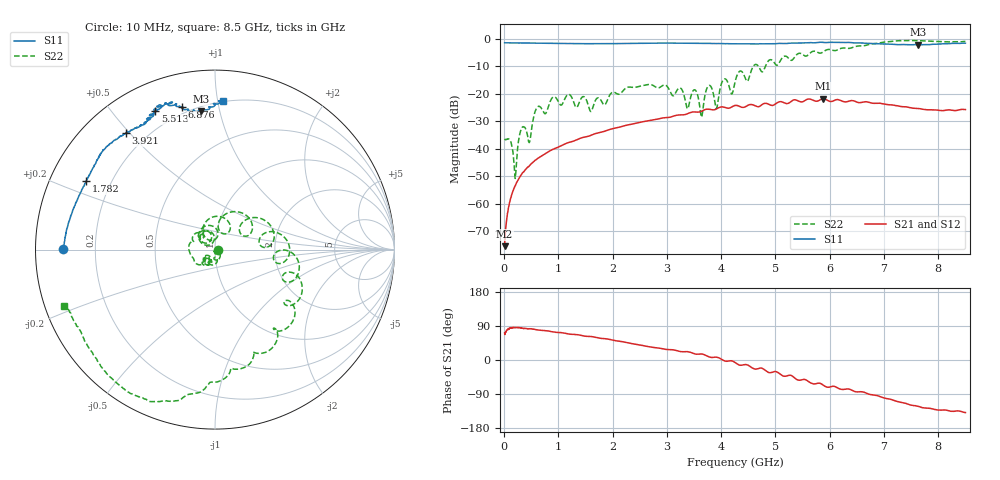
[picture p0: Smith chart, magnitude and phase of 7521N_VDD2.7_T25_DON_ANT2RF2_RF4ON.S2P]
!Agilent Technologies,E5071C,MY46417908,A.11.23
!Date: Thu Jul 30 15:13:54 2020
!Data & Calibration Information:
!Freq	S11:SOLT2(ON)	S21:SOLT2(ON)	S12:SOLT2(ON)	S22:SOLT2(ON)
!PortZ  Port1:50+j0  Port2:50+j0
!Above PortZ is port z conversion or system Z0 setting when saving the data.
!When reading, reference impedance value at option line is always used.
# Hz S dB R 50
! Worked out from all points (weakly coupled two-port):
!   1601 points, 10 MHz to 8.5 GHz, reference 50 ohm
!   highest |S21| = -21.85 dB at 5.879 GHz (marker M1); lowest = -75.5 dB at 10 MHz (marker M2)
!   lowest |S11| = -2.2 dB at 7.624 GHz (marker M3), VSWR 7.90, Z = 11.3 + j43.8 ohm
!   |S11| at or under -10 dB: nowhere
!   |S22| runs from -50.9 to -0.6 dB; largest |S21 - S12| = 0.00077
!   S11 on the Smith chart (normalised r, x): 10 MHz: 0.08, +0.00; 1.782 GHz: 0.11, +0.25; 3.921 GHz: 0.13, +0.49; 5.513 GHz: 0.12, +0.65; 6.876 GHz: 0.17, +0.78; 8.5 GHz: 0.20, +1.04
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1e7  -1.45 179.9  -75.50 71.1  -75.74 70.6  -36.45 -13.7
2.063312e8  -1.52 176.8  -53.48 85.7  -53.52 86.2  -50.86 109.4
3.389875e8  -1.54 174.9  -48.87 84.1  -48.86 84.0  -32.16 -58.3
4.663375e8  -1.57 173.0  -46.23 82.4  -46.23 82.9  -37.73 -67.2
5.989938e8  -1.61 170.9  -43.83 79.9  -43.81 80.0  -25.27 -63.1
9.067562e8  -1.69 166.1  -40.20 74.0  -40.20 74.1  -21.20 -99.1
1.426769e9  -1.79 157.9  -36.08 64.7  -36.09 64.6  -21.52 -121.8
1.782288e9  -1.79 152.0  -34.04 57.2  -34.05 57.1  -22.32 -134.3
2.843538e9  -1.59 140.0  -29.20 31.6  -29.19 31.6  -17.91 159.2
3.517431e9  -1.63 133.0  -26.66 15.9  -26.66 15.9  -18.62 120.4
3.639475e9  -1.68 131.9  -26.37 15.9  -26.36 15.9  -28.55 125.6
3.78805e9  -1.69 129.8  -25.70 7.6  -25.70 7.7  -16.99 110.7
3.920706e9  -1.76 127.4  -25.47 7.4  -25.46 7.3  -25.21 112.1
4.04275e9  -1.78 126.5  -24.86 -1.0  -24.87 -1.0  -14.86 95.2
4.255e9  -1.82 123.4  -24.29 -6.6  -24.29 -6.5  -15.81 81.5
5.512581e9  -1.51 113.2  -22.86 -51.3  -22.88 -51.3  -5.90 -37.9
5.671769e9  -1.45 113.6  -22.17 -61.9  -22.16 -61.8  -4.73 -40.2
5.878712e9  -1.34 112.1  -21.85 -66.0  -21.84 -65.8  -4.81 -52.9
6.876288e9  -1.79 103.1  -23.48 -93.9  -23.48 -94.0  -1.72 -100.4
7.088538e9  -1.98 100.8  -24.03 -102.7  -24.04 -102.8  -1.08 -106.9
7.624469e9  -2.21 95.9  -25.37 -122.0  -25.36 -122.1  -0.70 -126.8
8.5e9  -1.62 86.8  -25.79 -138.7  -25.87 -139.3  -0.96 -159.6
